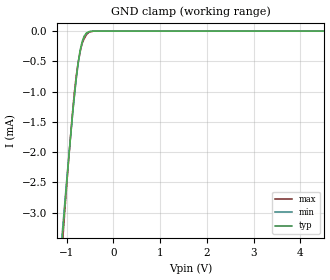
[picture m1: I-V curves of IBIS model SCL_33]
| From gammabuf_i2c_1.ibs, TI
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|   Input SCL model 3V
[Model]   SCL_33
Model_type   Input
|Signals   SCL
Vinl = 0.99
Vinh = 1.5
|   typ   min   max
C_comp   6.1203700e-12   7.3057800e-12  5.0777520e-12
[Voltage Range]   3.3   3   3.6
[Temperature Range]   27   85   -40
[Power Clamp Reference]   3.3   3   3.6
[GND Clamp Reference]   0   0   0
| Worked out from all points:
|   GND clamp passes 1 mA (typ) near -0.82 V on its own axis
[GND Clamp]
|   Voltage   I(typ)   I(min)   I(max)
-3.3V     -27.23mA   -25.53mA   -29.55mA
-1.089V   -3.407mA   -3.305mA   -3.537mA
-1.038V   -2.904mA   -2.833mA   -2.983mA
-953.4mV  -2.106mA   -2.077mA   -2.109mA
-884.3mV  -1.493mA   -1.492mA   -1.443mA
-830.2mV  -1.052mA   -1.065mA   -991.1uA
-787.6mV  -744.5uA   -764.1uA   -708.2uA
-720mV    -363.2uA   -388.6uA   -390.1uA
-669.2mV  -182uA     -203.8uA   -218.7uA
-612.2mV  -70.73uA   -80.97uA   -112.1uA
-519.9mV  -9.237uA   -11.35uA   -21.65uA
6.59V     0A         0A         0A
[POWER Clamp]
|   Voltage   I(typ)   I(min)   I(max)
-3.3V     0A         0A         0A
0V        0A         0A         0A
6.6V      0A         0A         0A
